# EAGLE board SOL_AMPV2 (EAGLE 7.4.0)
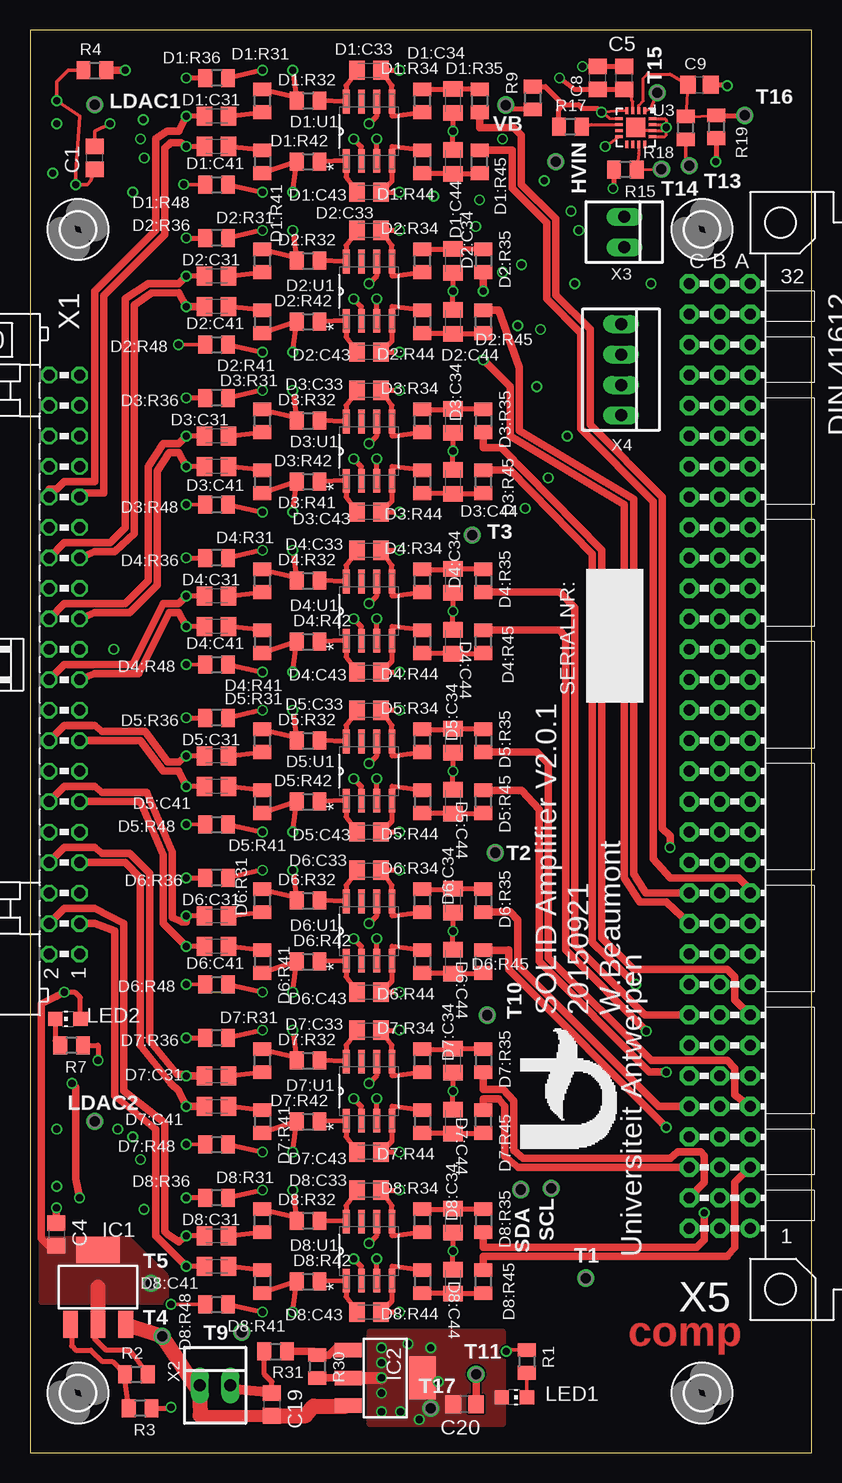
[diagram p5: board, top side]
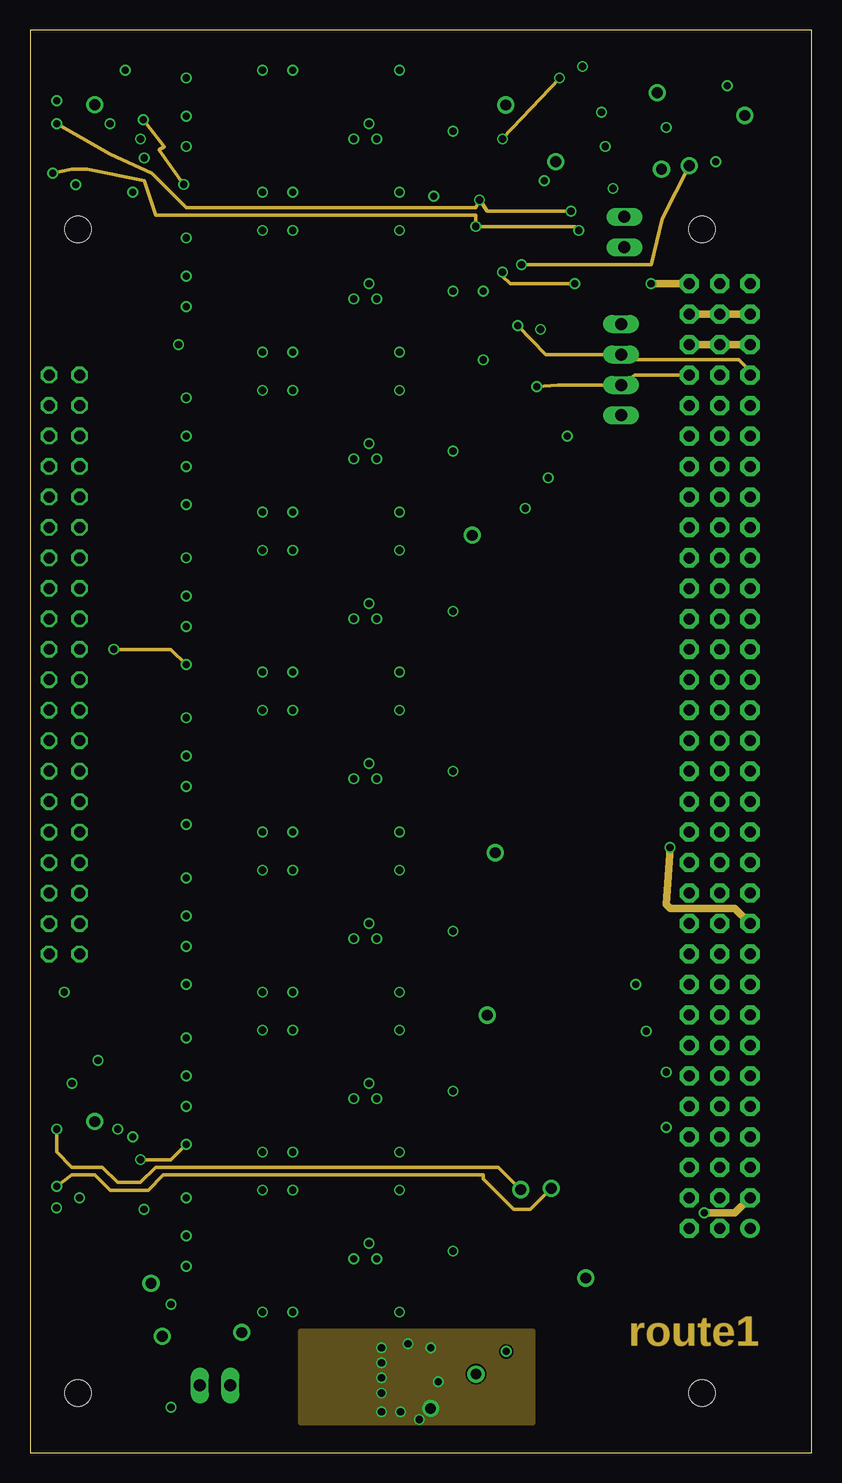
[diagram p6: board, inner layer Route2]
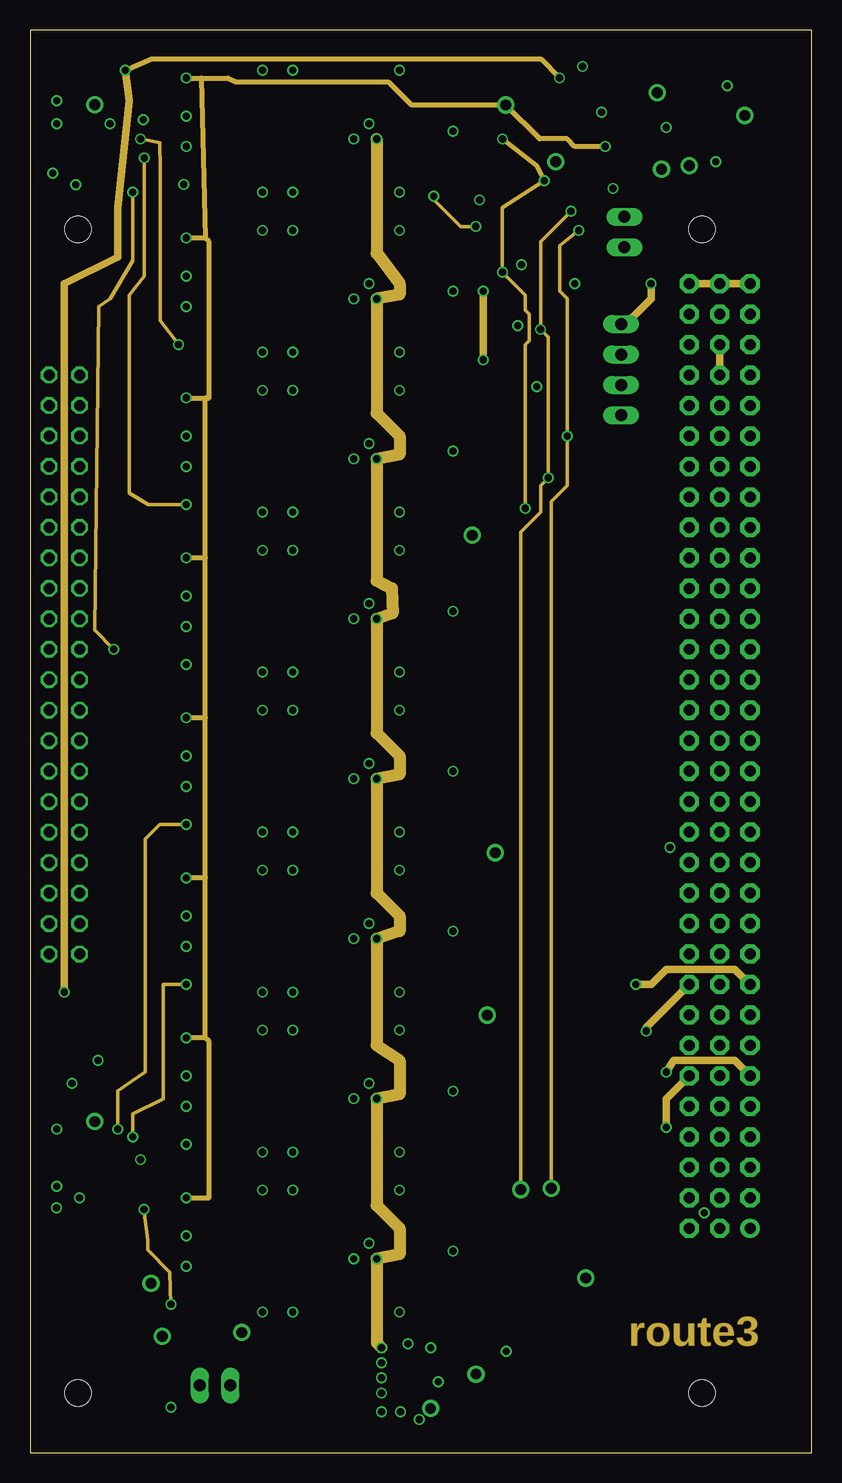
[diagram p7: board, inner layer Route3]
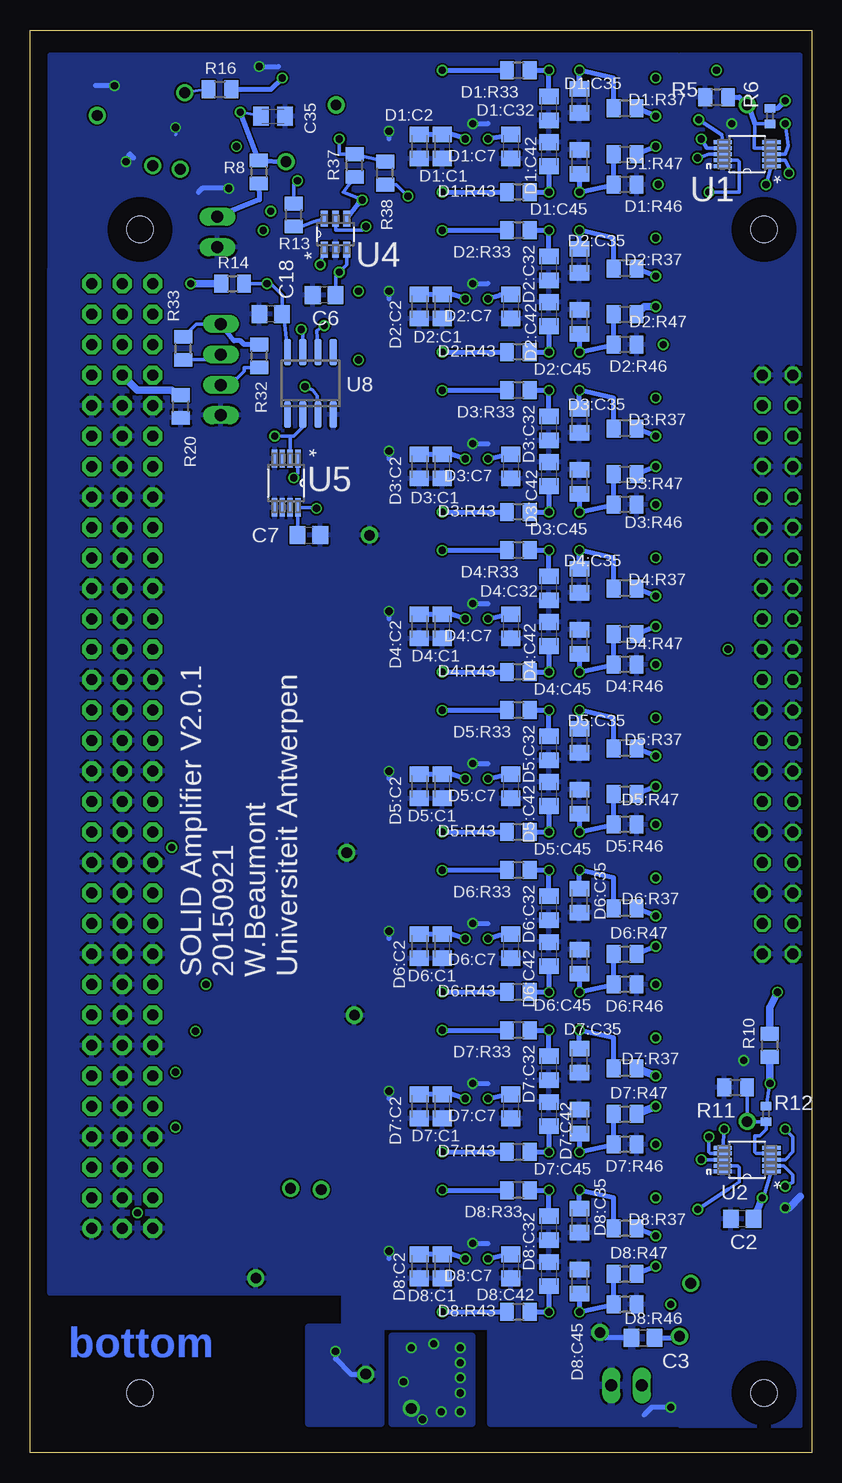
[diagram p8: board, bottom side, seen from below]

Size 65.15 x 118.62 mm. Coordinates in mm from the lower left corner, seen from the top.
Outline: 0,0 65.15,0 65.15,118.62 0,118.62 0,0
Copper layers (1+2*3+16): Top 0.018mm / dielectric 0.36mm / Route2 0.035mm / dielectric 0.71mm / Route3 0.035mm / dielectric 0.36mm / Bottom 0.018mm
Design rules "eC_4Layer_PClass6_BaseCopperO18-I35_eCDefault": minimum track width 0.15mm, minimum drill 0.35mm, track to track 0.15mm, track to pad 0.15mm, pad to pad 0.15mm, via to via 0.15mm, smd to smd 0mil, copper to edge 0.25mm, drill to drill 0.35mm, minimum pad ring 0.175mm, minimum via ring 0.125mm, stop-mask expansion 0mil, vias tented up to drill 0.45mm, thermal gap 0.2mm

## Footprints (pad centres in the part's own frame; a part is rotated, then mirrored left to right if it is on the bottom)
C0805 = smd 1.3 x 1.5: 1 -0.95,0; 2 0.95,0
C0805K = smd 1.3 x 1.6: 1 -1,0; 2 1,0
R0805H = smd 1.143 x 1.5: 1 -0.95,0; 2 0.95,0
SOIC127P600X175-8N = smd 1.981 x 0.559: 1 -2.464,1.905; 2 -2.464,0.635; 3 -2.464,-0.635; 4 -2.464,-1.905; 5 2.464,-1.905; 6 2.464,-0.635; 7 2.464,0.635; 8 2.464,1.905
2,1 = hole 2.2: 0,0
UA_P1-13 = drill 0.9 pad 1.422: TP 0,0
SOT223 = smd 1.219 x 2.235: 1 -2.311,-3.099; 2 0,-3.099; 3 2.311,-3.099 | smd 3.6 x 2.2: 4 0,3.099
CHIP-LED0805 = smd 1.2 x 1.2: A 0,-1.05; C 0,1.05
R0402 = smd 0.7 x 0.9: 1 -0.65,0; 2 0.65,0
SOP50P490X110-10N = smd 1.524 x 0.33: 1 -2.032,0.991; 2 -2.032,0.508; 3 -2.032,0; 4 -2.032,-0.508; 5 -2.032,-0.991; 6 2.032,-0.991; 7 2.032,-0.508; 8 2.032,0; 9 2.032,0.508; 10 2.032,0.991
LFCSP_LQ-16_MANSOL = smd 0.61 x 0.25: 1 -1.405,0.75; 2 -1.405,0.25; 3 -1.405,-0.25; 4 -1.405,-0.75; 9 1.405,-0.75; 10 1.405,-0.25; 11 1.405,0.25; 12 1.405,0.75 | smd 0.25 x 0.61: 5 -0.75,-1.405; 6 -0.25,-1.405; 7 0.25,-1.405; 8 0.75,-1.405; 13 0.75,1.405; 14 0.25,1.405; 15 -0.25,1.405; 16 -0.75,1.405 | smd 1.6 x 1.6: EXP 0,0
SOT95P270X145-6N = smd 1.321 x 0.559: 1 -1.295,0.94; 2 -1.295,0; 3 -1.295,-0.94; 4 1.295,-0.94; 5 1.295,0; 6 1.295,0.94
SOP65P490X110-8N = smd 1.524 x 0.457: 1 -2.032,0.965; 2 -2.032,0.33; 3 -2.032,-0.33; 4 -2.032,-0.965; 5 2.032,-0.965; 6 2.032,-0.33; 7 2.032,0.33; 8 2.032,0.965
SO8 = smd 0.6 x 2.2: 1 -1.905,-2.6; 2 -0.635,-2.6; 3 0.635,-2.6; 4 1.905,-2.6; 5 1.905,2.6; 6 0.635,2.6; 7 -0.635,2.6; 8 -1.905,2.6
ML40L = drill 0.914 octagon: 1 -24.13,-1.27; 2 -24.13,1.27; 3 -21.59,-1.27; 4 -21.59,1.27; 5 -19.05,-1.27; 6 -19.05,1.27; 7 -16.51,-1.27; 8 -16.51,1.27; 9 -13.97,-1.27; 10 -13.97,1.27; 11 -11.43,-1.27; 12 -11.43,1.27; 13 -8.89,-1.27; 14 -8.89,1.27; 15 -6.35,-1.27; 16 -6.35,1.27; 17 -3.81,-1.27; 18 -3.81,1.27; 19 -1.27,-1.27; 20 -1.27,1.27; 21 1.27,-1.27; 22 1.27,1.27; 23 3.81,-1.27; 24 3.81,1.27; 25 6.35,-1.27; 26 6.35,1.27; 27 8.89,-1.27; 28 8.89,1.27; 29 11.43,-1.27; 30 11.43,1.27; 31 13.97,-1.27; 32 13.97,1.27; 33 16.51,-1.27; 34 16.51,1.27; 35 19.05,-1.27; 36 19.05,1.27; 37 21.59,-1.27; 38 21.59,1.27; 39 24.13,-1.27; 40 24.13,1.27
22-23-2021 = drill 1 long: 1 -1.27,0; 2 1.27,0
22-23-2041 = drill 1 long: 1 -3.81,0; 2 -1.27,0; 3 1.27,0; 4 3.81,0
DIN41612_96RC = drill 0.914 pad 1.6: A1 2.54,-39.37 | drill 0.914 pad 1.6 octagon: A2 2.54,-36.83; A3 2.54,-34.29; A4 2.54,-31.75; A5 2.54,-29.21; A6 2.54,-26.67; A7 2.54,-24.13; A8 2.54,-21.59; A9 2.54,-19.05; A10 2.54,-16.51; A11 2.54,-13.97; A12 2.54,-11.43; A13 2.54,-8.89; A14 2.54,-6.35; A15 2.54,-3.81; A16 2.54,-1.27; A17 2.54,1.27; A18 2.54,3.81; A19 2.54,6.35; A20 2.54,8.89; A21 2.54,11.43; A22 2.54,13.97; A23 2.54,16.51; A24 2.54,19.05; A25 2.54,21.59; A26 2.54,24.13; A27 2.54,26.67; A28 2.54,29.21; A29 2.54,31.75; A30 2.54,34.29; A31 2.54,36.83; A32 2.54,39.37; B1 0,-39.37; B2 0,-36.83; B3 0,-34.29; B4 0,-31.75; B5 0,-29.21; B6 0,-26.67; B7 0,-24.13; B8 0,-21.59; B9 0,-19.05; B10 0,-16.51; B11 0,-13.97; B12 0,-11.43; B13 0,-8.89; B14 0,-6.35; B15 0,-3.81; B16 0,-1.27; B17 0,1.27; B18 0,3.81; B19 0,6.35; B20 0,8.89; B21 0,11.43; B22 0,13.97; B23 0,16.51; B24 0,19.05; B25 0,21.59; B26 0,24.13; B27 0,26.67; B28 0,29.21; B29 0,31.75; B30 0,34.29; B31 0,36.83; B32 0,39.37; C1 -2.54,-39.37; C2 -2.54,-36.83; C3 -2.54,-34.29; C4 -2.54,-31.75; C5 -2.54,-29.21; C6 -2.54,-26.67; C7 -2.54,-24.13; C8 -2.54,-21.59; C9 -2.54,-19.05; C10 -2.54,-16.51; C11 -2.54,-13.97; C12 -2.54,-11.43; C13 -2.54,-8.89; C14 -2.54,-6.35; C15 -2.54,-3.81; C16 -2.54,-1.27; C17 -2.54,1.27; C18 -2.54,3.81; C19 -2.54,6.35; C20 -2.54,8.89; C21 -2.54,11.43; C22 -2.54,13.97; C23 -2.54,16.51; C24 -2.54,19.05; C25 -2.54,21.59; C26 -2.54,24.13; C27 -2.54,26.67; C28 -2.54,29.21; C29 -2.54,31.75; C30 -2.54,34.29; C31 -2.54,36.83; C32 -2.54,39.37

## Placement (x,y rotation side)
C1  10u  [C0805]  5.4,107.95 90 top
C2  10u  [C0805]  5.79,19.51 180 bottom
C3  10uF  [C0805]  14.06,9.59 0 bottom
C4  10uF  [C0805]  2.21,18.22 270 top
C5  10n  [C0805]  49.53,114.62 90 top
C6  10n  [C0805]  40.64,96.52 180 bottom
C7  10n  [C0805]  41.91,76.52 0 bottom
C8  100n  [C0805]  47.31,114.62 90 top
C9  10n  [C0805]  55.78,114.05 0 top
C18  10n  [C0805]  45.09,94.93 180 bottom
C19  10uF  [C0805]  20.16,4.05 270 top
C20  10uF  [C0805]  36.22,4.05 180 top
C35  100nF /100V  [C0805K]  44.9,111.42 0 bottom
D1:C1  100n  [C0805K]  30.8,108.9 90 bottom
D1:C2  10n  [C0805K]  32.7,108.9 90 bottom
D1:C7  10n  [C0805K]  25.08,108.9 270 bottom
D1:C31  4.4n/100V  [C0805K]  15.56,111.44 180 top
D1:C32  152p  [C0805K]  21.91,112.08 90 bottom
D1:C33  21p  [C0805K]  28.26,115.25 0 top
D1:C34  x  [C0805K]  35.24,112.71 90 top
D1:C35  100nF /100V  [C0805K]  19.37,112.71 270 bottom
D1:C41  4.4n  [C0805K]  15.56,108.9 180 top
D1:C42  152p  [C0805K]  21.91,108.27 270 bottom
D1:C43  21p  [C0805K]  28.26,105.09 0 top
D1:C44  x  [C0805K]  35.24,107.63 270 top
D1:C45  100nF /100V  [C0805K]  19.37,107.63 90 bottom
D1:R31  27  [R0805H]  19.37,112.71 90 top
D1:R32  24  [R0805H]  23.18,112.71 0 top
D1:R33  3K  [R0805H]  24.45,115.25 180 bottom
D1:R34  1  [R0805H]  32.7,112.71 90 top
D1:R35  1  [R0805H]  37.47,112.71 270 top
D1:R36  10K  [R0805H]  15.56,114.62 180 top
D1:R37  100K  [R0805H]  15.56,112.08 180 bottom
D1:R41  27  [R0805H]  19.37,107.63 270 top
D1:R42  24  [R0805H]  23.18,107.63 0 top
D1:R43  3K  [R0805H]  24.45,105.09 180 bottom
D1:R44  1  [R0805H]  32.7,107.63 270 top
D1:R45  1  [R0805H]  37.47,107.63 90 top
D1:R46  10K  [R0805H]  15.56,105.73 180 bottom
D1:R47  100K  [R0805H]  15.56,108.27 0 bottom
D1:R48  470  [R0805H]  15.56,105.73 0 top
D1:U1  AD8132ARZ  [SOIC127P600X175-8N]  28.26,110.17 90 top
D2:C1  100n  [C0805K]  30.8,95.57 90 bottom
D2:C2  10n  [C0805K]  32.7,95.57 90 bottom
D2:C7  10n  [C0805K]  25.08,95.57 270 bottom
D2:C31  4.4n/100V  [C0805K]  15.56,98.11 180 top
D2:C32  152p  [C0805K]  21.91,98.74 90 bottom
D2:C33  21p  [C0805K]  28.26,101.92 0 top
D2:C34  x  [C0805K]  35.24,99.38 90 top
D2:C35  100nF /100V  [C0805K]  19.37,99.38 270 bottom
D2:C41  4.4n  [C0805K]  15.56,95.57 180 top
D2:C42  152p  [C0805K]  21.91,94.93 270 bottom
D2:C43  21p  [C0805K]  28.26,91.76 0 top
D2:C44  x  [C0805K]  35.24,94.3 270 top
D2:C45  100nF /100V  [C0805K]  19.37,94.3 90 bottom
D2:R31  27  [R0805H]  19.37,99.38 90 top
D2:R32  24  [R0805H]  23.18,99.38 0 top
D2:R33  3K  [R0805H]  24.45,101.92 180 bottom
D2:R34  1  [R0805H]  32.7,99.38 90 top
D2:R35  1  [R0805H]  37.78,99.38 270 top
D2:R36  10K  [R0805H]  15.56,101.28 180 top
D2:R37  100K  [R0805H]  15.56,98.74 180 bottom
D2:R41  27  [R0805H]  19.37,94.3 270 top
D2:R42  24  [R0805H]  23.18,94.3 0 top
D2:R43  3K  [R0805H]  24.45,91.76 180 bottom
D2:R44  1  [R0805H]  32.7,94.3 270 top
D2:R45  1  [R0805H]  37.78,94.3 90 top
D2:R46  10K  [R0805H]  15.56,92.39 180 bottom
D2:R47  100K  [R0805H]  15.56,94.93 0 bottom
D2:R48  470  [R0805H]  15.56,92.39 0 top
D2:U1  AD8132ARZ  [SOIC127P600X175-8N]  28.26,96.84 90 top
D3:C1  100n  [C0805K]  30.8,82.23 90 bottom
D3:C2  10n  [C0805K]  32.7,82.23 90 bottom
D3:C7  10n  [C0805K]  25.08,82.23 270 bottom
D3:C31  4.4n/100V  [C0805K]  15.56,84.77 180 top
D3:C32  152p  [C0805K]  21.91,85.41 90 bottom
D3:C33  21p  [C0805K]  28.26,88.58 0 top
D3:C34  x  [C0805K]  35.24,86.04 90 top
D3:C35  100nF /100V  [C0805K]  19.37,86.04 270 bottom
D3:C41  4.4n  [C0805K]  15.56,82.23 180 top
D3:C42  152p  [C0805K]  21.91,81.6 270 bottom
D3:C43  21p  [C0805K]  28.26,78.42 0 top
D3:C44  x  [C0805K]  35.24,80.96 270 top
D3:C45  100nF /100V  [C0805K]  19.37,80.96 90 bottom
D3:R31  27  [R0805H]  19.37,86.04 90 top
D3:R32  24  [R0805H]  23.18,86.04 0 top
D3:R33  3K  [R0805H]  24.45,88.58 180 bottom
D3:R34  1  [R0805H]  32.7,86.04 90 top
D3:R35  1  [R0805H]  37.78,86.04 270 top
D3:R36  10K  [R0805H]  15.56,87.95 180 top
D3:R37  100K  [R0805H]  15.56,85.41 180 bottom
D3:R41  27  [R0805H]  19.37,80.96 270 top
D3:R42  24  [R0805H]  23.18,80.96 0 top
D3:R43  3K  [R0805H]  24.45,78.42 180 bottom
D3:R44  1  [R0805H]  32.7,80.96 270 top
D3:R45  1  [R0805H]  37.78,80.96 90 top
D3:R46  10K  [R0805H]  15.56,79.06 180 bottom
D3:R47  100K  [R0805H]  15.56,81.6 0 bottom
D3:R48  470  [R0805H]  15.56,79.06 0 top
D3:U1  AD8132ARZ  [SOIC127P600X175-8N]  28.26,83.5 90 top
D4:C1  100n  [C0805K]  30.8,68.9 90 bottom
D4:C2  10n  [C0805K]  32.7,68.9 90 bottom
D4:C7  10n  [C0805K]  25.08,68.9 270 bottom
D4:C31  4.4n/100V  [C0805K]  15.56,71.44 180 top
D4:C32  152p  [C0805K]  21.91,72.07 90 bottom
D4:C33  21p  [C0805K]  28.26,75.25 0 top
D4:C34  x  [C0805K]  35.24,72.71 90 top
D4:C35  100nF /100V  [C0805K]  19.37,72.71 270 bottom
D4:C41  4.4n  [C0805K]  15.56,68.9 180 top
D4:C42  152p  [C0805K]  21.91,68.26 270 bottom
D4:C43  21p  [C0805K]  28.26,65.09 0 top
D4:C44  x  [C0805K]  35.24,67.63 270 top
D4:C45  100nF /100V  [C0805K]  19.37,67.63 90 bottom
D4:R31  27  [R0805H]  19.37,72.71 90 top
D4:R32  24  [R0805H]  23.18,72.71 0 top
D4:R33  3K  [R0805H]  24.45,75.25 180 bottom
D4:R34  1  [R0805H]  32.7,72.71 90 top
D4:R35  1  [R0805H]  37.78,72.71 270 top
D4:R36  10K  [R0805H]  15.56,74.61 180 top
D4:R37  100K  [R0805H]  15.56,72.07 180 bottom
D4:R41  27  [R0805H]  19.37,67.63 270 top
D4:R42  24  [R0805H]  23.18,67.63 0 top
D4:R43  3K  [R0805H]  24.45,65.09 180 bottom
D4:R44  1  [R0805H]  32.7,67.63 270 top
D4:R45  1  [R0805H]  37.78,67.63 90 top
D4:R46  10K  [R0805H]  15.56,65.72 180 bottom
D4:R47  100K  [R0805H]  15.56,68.26 0 bottom
D4:R48  470  [R0805H]  15.56,65.72 0 top
D4:U1  AD8132ARZ  [SOIC127P600X175-8N]  28.26,70.17 90 top
D5:C1  100n  [C0805K]  30.8,55.56 90 bottom
D5:C2  10n  [C0805K]  32.7,55.56 90 bottom
D5:C7  10n  [C0805K]  25.08,55.56 270 bottom
D5:C31  4.4n/100V  [C0805K]  15.56,58.1 180 top
D5:C32  152p  [C0805K]  21.91,58.74 90 bottom
D5:C33  21p  [C0805K]  28.26,61.91 0 top
D5:C34  x  [C0805K]  35.24,59.37 90 top
D5:C35  100nF /100V  [C0805K]  19.37,59.37 270 bottom
D5:C41  4.4n  [C0805K]  15.56,55.56 180 top
D5:C42  152p  [C0805K]  21.91,54.93 270 bottom
D5:C43  21p  [C0805K]  28.26,51.75 0 top
D5:C44  x  [C0805K]  35.24,54.29 270 top
D5:C45  100nF /100V  [C0805K]  19.37,54.29 90 bottom
D5:R31  27  [R0805H]  19.37,59.37 90 top
D5:R32  24  [R0805H]  23.18,59.37 0 top
D5:R33  3K  [R0805H]  24.45,61.91 180 bottom
D5:R34  1  [R0805H]  32.7,59.37 90 top
D5:R35  1  [R0805H]  37.78,59.37 270 top
D5:R36  10K  [R0805H]  15.56,61.28 180 top
D5:R37  100K  [R0805H]  15.56,58.74 180 bottom
D5:R41  27  [R0805H]  19.37,54.29 270 top
D5:R42  24  [R0805H]  23.18,54.29 0 top
D5:R43  3K  [R0805H]  24.45,51.75 180 bottom
D5:R44  1  [R0805H]  32.7,54.29 270 top
D5:R45  1  [R0805H]  37.78,54.29 90 top
D5:R46  10K  [R0805H]  15.56,52.39 180 bottom
D5:R47  100K  [R0805H]  15.56,54.93 0 bottom
D5:R48  470  [R0805H]  15.56,52.39 0 top
D5:U1  AD8132ARZ  [SOIC127P600X175-8N]  28.26,56.83 90 top
D6:C1  100n  [C0805K]  30.8,42.23 90 bottom
D6:C2  10n  [C0805K]  32.7,42.23 90 bottom
D6:C7  10n  [C0805K]  25.08,42.23 270 bottom
D6:C31  4.4n/100V  [C0805K]  15.56,44.77 180 top
D6:C32  152p  [C0805K]  21.91,45.4 90 bottom
D6:C33  21p  [C0805K]  28.26,48.58 0 top
D6:C34  x  [C0805K]  35.24,46.04 90 top
D6:C35  100nF /100V  [C0805K]  19.37,46.04 270 bottom
D6:C41  4.4n  [C0805K]  15.56,42.23 180 top
D6:C42  152p  [C0805K]  21.91,41.59 270 bottom
D6:C43  21p  [C0805K]  28.26,38.42 0 top
D6:C44  x  [C0805K]  35.24,40.96 270 top
D6:C45  100nF /100V  [C0805K]  19.37,40.96 90 bottom
D6:R31  27  [R0805H]  19.37,46.04 90 top
D6:R32  24  [R0805H]  23.18,46.04 0 top
D6:R33  3K  [R0805H]  24.45,48.58 180 bottom
D6:R34  1  [R0805H]  32.7,46.04 90 top
D6:R35  1  [R0805H]  37.78,46.04 270 top
D6:R36  10K  [R0805H]  15.56,47.94 180 top
D6:R37  100K  [R0805H]  15.56,45.4 180 bottom
D6:R41  27  [R0805H]  19.37,40.96 270 top
D6:R42  24  [R0805H]  23.18,40.96 0 top
D6:R43  3K  [R0805H]  24.45,38.42 180 bottom
D6:R44  1  [R0805H]  32.7,40.96 270 top
D6:R45  1  [R0805H]  37.78,40.96 90 top
D6:R46  10K  [R0805H]  15.56,39.05 180 bottom
D6:R47  100K  [R0805H]  15.56,41.59 0 bottom
D6:R48  470  [R0805H]  15.56,39.05 0 top
D6:U1  AD8132ARZ  [SOIC127P600X175-8N]  28.26,43.5 90 top
D7:C1  100n  [C0805K]  30.8,28.89 90 bottom
D7:C2  10n  [C0805K]  32.7,28.89 90 bottom
D7:C7  10n  [C0805K]  25.08,28.89 270 bottom
D7:C31  4.4n/100V  [C0805K]  15.56,31.43 180 top
D7:C32  152p  [C0805K]  21.91,32.07 90 bottom
D7:C33  21p  [C0805K]  28.26,35.24 0 top
D7:C34  x  [C0805K]  35.24,32.7 90 top
D7:C35  100nF /100V  [C0805K]  19.37,32.7 270 bottom
D7:C41  4.4n  [C0805K]  15.56,28.89 180 top
D7:C42  152p  [C0805K]  21.91,28.26 270 bottom
D7:C43  21p  [C0805K]  28.26,25.08 0 top
D7:C44  x  [C0805K]  35.24,27.62 270 top
D7:C45  100nF /100V  [C0805K]  19.37,27.62 90 bottom
D7:R31  27  [R0805H]  19.37,32.7 90 top
D7:R32  24  [R0805H]  23.18,32.7 0 top
D7:R33  3K  [R0805H]  24.45,35.24 180 bottom
D7:R34  1  [R0805H]  32.7,32.7 90 top
D7:R35  1  [R0805H]  37.78,32.7 270 top
D7:R36  10K  [R0805H]  15.56,34.61 180 top
D7:R37  100K  [R0805H]  15.56,32.07 180 bottom
D7:R41  27  [R0805H]  19.37,27.62 270 top
D7:R42  24  [R0805H]  23.18,27.62 0 top
D7:R43  3K  [R0805H]  24.45,25.08 180 bottom
D7:R44  1  [R0805H]  32.7,27.62 270 top
D7:R45  1  [R0805H]  37.78,27.62 90 top
D7:R46  10K  [R0805H]  15.56,25.72 180 bottom
D7:R47  100K  [R0805H]  15.56,28.26 0 bottom
D7:R48  470  [R0805H]  15.56,25.72 0 top
D7:U1  AD8132ARZ  [SOIC127P600X175-8N]  28.26,30.16 90 top
D8:C1  100n  [C0805K]  30.8,15.56 90 bottom
D8:C2  10n  [C0805K]  32.7,15.56 90 bottom
D8:C7  10n  [C0805K]  25.08,15.56 270 bottom
D8:C31  4.4n/100V  [C0805K]  15.56,18.1 180 top
D8:C32  152p  [C0805K]  21.91,18.73 90 bottom
D8:C33  21p  [C0805K]  28.26,21.91 0 top
D8:C34  x  [C0805K]  35.24,19.37 90 top
D8:C35  100nF /100V  [C0805K]  19.37,19.37 270 bottom
D8:C41  4.4n  [C0805K]  15.56,15.56 180 top
D8:C42  152p  [C0805K]  21.91,14.92 270 bottom
D8:C43  21p  [C0805K]  28.26,11.75 0 top
D8:C44  x  [C0805K]  35.24,14.29 270 top
D8:C45  100nF /100V  [C0805K]  19.37,14.29 90 bottom
D8:R31  27  [R0805H]  19.37,19.37 90 top
D8:R32  24  [R0805H]  23.18,19.37 0 top
D8:R33  3K  [R0805H]  24.45,21.91 180 bottom
D8:R34  1  [R0805H]  32.7,19.37 90 top
D8:R35  1  [R0805H]  37.78,19.37 270 top
D8:R36  10K  [R0805H]  15.56,21.27 180 top
D8:R37  100K  [R0805H]  15.56,18.73 180 bottom
D8:R41  27  [R0805H]  19.37,14.29 270 top
D8:R42  24  [R0805H]  23.18,14.29 0 top
D8:R43  3K  [R0805H]  24.45,11.75 180 bottom
D8:R44  1  [R0805H]  32.7,14.29 270 top
D8:R45  1  [R0805H]  37.78,14.29 90 top
D8:R46  10K  [R0805H]  15.56,12.38 180 bottom
D8:R47  100K  [R0805H]  15.56,14.92 0 bottom
D8:R48  470  [R0805H]  15.56,12.38 0 top
D8:U1  AD8132ARZ  [SOIC127P600X175-8N]  28.26,16.83 90 top
H1  [2,1]  4,5 0 top
H2  [2,1]  56,5 0 top
H3  [2,1]  4,102 0 top
H4  [2,1]  56,102 0 top
HVIN  UA_TPPAD1-13  [UA_P1-13]  43.81,107.63 0 top
IC1  LM1117  [SOT223]  5.67,13.82 0 top
IC2  LM1117  [SOT223]  29.61,6.26 270 top
LDAC1  UA_TPPAD1-13  [UA_P1-13]  5.4,112.39 0 top
LDAC2  UA_TPPAD1-13  [UA_P1-13]  5.4,27.62 0 top
LED1  HSMY-C170  [CHIP-LED0805]  40.36,4.64 270 top
LED2  HSMY-C170  [CHIP-LED0805]  3.15,36.18 90 top
M1  [UA]  45.09,29.21 90 top
R1  1K  [R0805H]  41.4,7.63 270 top
R2  330E  [R0805H]  8.86,6.57 0 top
R3  1K  [R0805H]  9.17,3.73 180 top
R4  10E  [R0805H]  5.4,115.25 0 top
R5  4.7K  [R0805H]  7.94,113.03 0 bottom
R6  NC  [R0402]  3.49,111.44 90 bottom
R7  1K  [R0805H]  3.47,33.97 180 top
R8  1K  [R0805H]  46.09,106.79 270 bottom
R9  NC  [R0805H]  41.91,112.95 90 top
R10  10  [R0805H]  3.49,33.97 90 bottom
R11  4.7K  [R0805H]  6.35,30.48 0 bottom
R12  NC  [R0402]  3.81,28.26 90 bottom
R13  4K7  [R0805H]  43.18,103.19 90 bottom
R14  NC  [R0805H]  48.26,97.47 0 bottom
R15  27K  [R0805H]  49.62,106.96 180 top
R16  1K  [R0805H]  49.32,113.67 0 bottom
R17  NC  [R0805H]  45.03,110.57 0 top
R18  1K  [R0805H]  54.65,110.45 90 top
R19  2.4K  [R0805H]  57.19,110.54 270 top
R20  0  [R0805H]  52.58,87.24 90 bottom
R30  330E  [R0805H]  23.94,7.2 270 top
R31  1K  [R0805H]  20.47,8.46 0 top
R32  4K7  [R0805H]  46.04,91.44 90 bottom
R33  4K7  [R0805H]  52.39,92.08 90 bottom
R37  4K7  [R0805H]  38.1,107.31 90 bottom
R38  4K7  [R0805H]  35.56,106.68 90 bottom
SCL  UA_TPPAD1-13  [UA_P1-13]  43.44,22.06 0 top
SDA  UA_TPPAD1-13  [UA_P1-13]  40.89,21.95 0 top
T1  UA_TPPAD1-13  [UA_P1-13]  46.32,14.57 0 top
T2  UA_TPPAD1-13  [UA_P1-13]  38.76,50.04 0 top
T3  UA_TPPAD1-13  [UA_P1-13]  36.86,76.5 0 top
T4  UA_TPPAD1-13  [UA_P1-13]  11.03,9.73 0 top
T5  UA_TPPAD1-13  [UA_P1-13]  10.08,14.13 0 top
T9  UA_TPPAD1-13  [UA_P1-13]  17.65,10.04 0 top
T10  UA_TPPAD1-13  [UA_P1-13]  38.11,36.49 0 top
T11  UA_TPPAD1-13  [UA_P1-13]  37.17,6.57 0 top
T13  UA_TPPAD1-13  [UA_P1-13]  54.93,107.31 0 top
T14  UA_TPPAD1-13  [UA_P1-13]  52.62,107.01 0 top
T15  UA_TPPAD1-13  [UA_P1-13]  52.26,113.39 0 top
T16  UA_TPPAD1-13  [UA_P1-13]  59.56,111.5 0 top
T17  UA_TPPAD1-13  [UA_P1-13]  33.38,3.71 0 top
U1  MCP4728-E/UN  [SOP50P490X110-10N]  5.4,108.27 180 bottom
U2  MCP4728-E/UN  [SOP50P490X110-10N]  5.4,24.45 180 bottom
U3  ADL5317  [LFCSP_LQ-16_MANSOL]  50.48,110.49 270 top
U4  MCP4725A0T-E/CH  [SOT95P270X145-6N]  39.69,101.6 90 bottom
U5  MCP9808-E/MS  [SOP65P490X110-8N]  43.8,80.85 270 bottom
U8  P82B715TD  [SO8]  41.79,89.16 0 bottom
VB  UA_TPPAD1-13  [UA_P1-13]  39.64,112.37 0 top
X1  40pin  [ML40L]  2.86,65.72 90 top
X2  22-23-2021  [22-23-2021]  15.44,5.63 0 top
X3  22-23-2021  [22-23-2021]  49.53,101.78 270 top
X4  22-23-2041  [22-23-2041]  49.25,90.3 270 top
X5  DIN41612_ABC_96_R  [DIN41612_96RC]  57.47,58.1 0 top

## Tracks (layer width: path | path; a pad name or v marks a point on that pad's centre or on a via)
BIASSET
  Top 0.254: U3.2 50.72,112.32 51.12,112.71 51.12,114.62 51.44,114.94 53.34,114.94 C9.1 R18.2 R19.1
  Top 0.406: R19.1 T16.TP
BIASTRSET  (via drill 0.6)
  Top 0.305: R18.1 54.65,107.6 T13.TP
  Route2 0.305: v40.96,99.06 51.75,99.06 52.7,102.87 T13.TP
  Bottom 0.305: U4.1 40.63,100.32 40.64,100.33 v40.96,99.06
D1:AOUT+  (via drill 0.6)
  Top 0.406: v30.8,105.09 D1:C43.2 30.16,106 D1:U1.4 30.16,108.9 D1:R44.1
  Bottom 0.406: v30.8,105.09 D1:R43.2
D1:AOUT-  (via drill 0.6)
  Top 0.406: D1:R34.1 30.16,111.44 D1:U1.5 30.16,113.98 D1:C33.2 v30.8,115.25
  Bottom 0.406: v30.8,115.25 D1:R33.2
D1:FB+  (via drill 0.6)
  Top 0.406: v21.91,115.25 D1:R32.1 D1:C32.2 D1:R31.2
  Bottom 0.406: D1:R33.1 v21.91,115.25 D1:C32.2
D1:FB-  (via drill 0.6)
  Top 0.406: v21.91,105.09 D1:R42.1 D1:R41.2
  Bottom 0.406: D1:R43.1 v21.91,105.09 D1:C42.2
D1:N$1
  Top 0.406: D1:R34.2 35.24,113.66 D1:C34.2 37.78,113.71 D1:R35.1
D1:N$2  (via drill 0.6)
  Top 0.406: D1:U1.2 27.62,108.9 v26.99,109.54
  Bottom 0.406: v26.99,109.54 25.35,109.86 D1:C7.1
D1:N$3
  Top 0.406: D1:R44.2 35.24,106.68 D1:C44.2 37.78,106.63 D1:R45.1
D1:N$4
  Top 0.406: D1:R42.2 D1:U1.1 26.35,106.36 D1:C43.1
D1:N$5
  Top 0.406: D1:C33.1 26.35,113.98 D1:U1.8 D1:R32.2
D1:N$10
  Top 0.406: D1:R41.1 D1:C41.1
D1:R31
  Top 0.406: D1:C31.1 D1:R31.1
D1:VB+  (via drill 0.6)
  Top 0.406: v19.37,115.25 D1:R36.1
  Bottom 0.406: D1:C35.1 v19.37,115.25 D1:R36.1 D1:R37.2
D1:VB-  (via drill 0.6)
  Top 0.406: D1:R46.2 v19.37,105.09
  Bottom 0.406: D1:R47.1 D1:R46.2 v19.37,105.09 D1:C45.1
D2:AOUT+  (via drill 0.6)
  Top 0.406: v30.8,91.76 D2:C43.2 30.16,92.66 D2:U1.4 30.16,95.57 D2:R44.1
  Bottom 0.406: v30.8,91.76 D2:R43.2
D2:AOUT-  (via drill 0.6)
  Top 0.406: D2:R34.1 30.16,98.11 D2:U1.5 30.16,100.65 D2:C33.2 v30.8,101.92
  Bottom 0.406: v30.8,101.92 D2:R33.2
D2:FB+  (via drill 0.6)
  Top 0.406: v21.91,101.92 D2:R32.1 D2:C32.2 D2:R31.2
  Bottom 0.406: D2:R33.1 v21.91,101.92 D2:C32.2
D2:FB-  (via drill 0.6)
  Top 0.406: v21.91,91.76 D2:R42.1 D2:R41.2
  Bottom 0.406: D2:R43.1 v21.91,91.76 D2:C42.2
D2:N$1
  Top 0.406: D2:R34.2 35.24,100.33 D2:C34.2 37.78,100.38 D2:R35.1
D2:N$2  (via drill 0.6)
  Top 0.406: D2:U1.2 27.62,95.57 v26.99,96.2
  Bottom 0.406: v26.99,96.2 25.99,96.52 D2:C7.1
D2:N$3
  Top 0.406: D2:R44.2 35.24,93.35 D2:C44.2 37.78,93.3 D2:R45.1
D2:N$4
  Top 0.406: D2:R42.2 D2:U1.1 26.35,93.03 D2:C43.1
D2:N$5
  Top 0.406: D2:C33.1 26.35,100.65 D2:U1.8 D2:R32.2
D2:N$10
  Top 0.406: D2:R41.1 D2:C41.1
D2:R31
  Top 0.406: D2:C31.1 D2:R31.1
D2:VB+  (via drill 0.6)
  Top 0.406: v19.37,101.92 D2:R36.1
  Bottom 0.406: D2:C35.1 v19.37,101.92 D2:R36.1 D2:R37.2
D2:VB-  (via drill 0.6)
  Top 0.406: D2:R46.2 v19.37,91.76
  Bottom 0.406: D2:R47.1 D2:R46.2 v19.37,91.76 D2:C45.1
D3:AOUT+  (via drill 0.6)
  Top 0.406: v30.8,78.42 D3:C43.2 30.16,79.33 D3:U1.4 30.16,82.23 D3:R44.1
  Bottom 0.406: v30.8,78.42 D3:R43.2
D3:AOUT-  (via drill 0.6)
  Top 0.406: D3:R34.1 30.16,84.77 D3:U1.5 30.16,87.31 D3:C33.2 v30.8,88.58
  Bottom 0.406: v30.8,88.58 D3:R33.2
D3:FB+  (via drill 0.6)
  Top 0.406: v21.91,88.58 D3:R32.1 D3:C32.2 D3:R31.2
  Bottom 0.406: D3:R33.1 v21.91,88.58 D3:C32.2
D3:FB-  (via drill 0.6)
  Top 0.406: v21.91,78.42 D3:R42.1 D3:R41.2
  Bottom 0.406: D3:R43.1 v21.91,78.42 D3:C42.2
D3:N$1
  Top 0.406: D3:R34.2 35.24,86.99 D3:C34.2 37.78,87.04 D3:R35.1
D3:N$2  (via drill 0.6)
  Top 0.406: D3:U1.2 27.62,82.23 v26.99,82.87
  Bottom 0.406: v26.99,82.87 25.67,83.19 D3:C7.1
D3:N$3
  Top 0.406: D3:R44.2 35.24,80.01 D3:C44.2 37.78,79.96 D3:R45.1
D3:N$4
  Top 0.406: D3:R42.2 D3:U1.1 26.35,79.69 D3:C43.1
D3:N$5
  Top 0.406: D3:C33.1 26.35,87.31 D3:U1.8 D3:R32.2
D3:N$10
  Top 0.406: D3:R41.1 D3:C41.1
D3:R31
  Top 0.406: D3:C31.1 D3:R31.1
D3:VB+  (via drill 0.6)
  Top 0.406: v19.37,88.58 D3:R36.1
  Bottom 0.406: D3:C35.1 v19.37,88.58 D3:R36.1 D3:R37.2
D3:VB-  (via drill 0.6)
  Top 0.406: D3:R46.2 v19.37,78.42
  Bottom 0.406: D3:R47.1 D3:R46.2 v19.37,78.42 D3:C45.1
D4:AOUT+  (via drill 0.6)
  Top 0.406: v30.8,65.09 D4:C43.2 30.16,65.99 D4:U1.4 30.16,68.9 D4:R44.1
  Bottom 0.406: v30.8,65.09 D4:R43.2
D4:AOUT-  (via drill 0.6)
  Top 0.406: D4:R34.1 30.16,71.44 D4:U1.5 30.16,73.98 D4:C33.2 v30.8,75.25
  Bottom 0.406: v30.8,75.25 D4:R33.2
D4:FB+  (via drill 0.6)
  Top 0.406: v21.91,75.25 D4:R32.1 D4:C32.2 D4:R31.2
  Bottom 0.406: D4:R33.1 v21.91,75.25 D4:C32.2
D4:FB-  (via drill 0.6)
  Top 0.406: v21.91,65.09 D4:R42.1 D4:R41.2
  Bottom 0.406: D4:R43.1 v21.91,65.09 D4:C42.2
D4:N$1
  Top 0.406: D4:R34.2 35.24,73.66 D4:C34.2 37.78,73.71 D4:R35.1
D4:N$2  (via drill 0.6)
  Top 0.406: D4:U1.2 27.62,68.9 v26.99,69.53
  Bottom 0.406: v26.99,69.53 25.67,69.85 D4:C7.1
D4:N$3
  Top 0.406: D4:R44.2 35.24,66.68 D4:C44.2 37.78,66.63 D4:R45.1
D4:N$4
  Top 0.406: D4:R42.2 D4:U1.1 26.35,66.36 D4:C43.1
D4:N$5
  Top 0.406: D4:C33.1 26.35,73.98 D4:U1.8 D4:R32.2
D4:N$10
  Top 0.406: D4:R41.1 D4:C41.1
D4:R31
  Top 0.406: D4:C31.1 D4:R31.1
D4:VB+  (via drill 0.6)
  Top 0.406: v19.37,75.25 D4:R36.1
  Bottom 0.406: D4:C35.1 v19.37,75.25 D4:R36.1 D4:R37.2
D4:VB-  (via drill 0.6)
  Top 0.406: D4:R46.2 v19.37,65.09
  Bottom 0.406: D4:R47.1 D4:R46.2 v19.37,65.09 D4:C45.1
D5:AOUT+  (via drill 0.6)
  Top 0.406: v30.8,51.75 D5:C43.2 30.16,52.66 D5:U1.4 30.16,55.56 D5:R44.1
  Bottom 0.406: v30.8,51.75 D5:R43.2
D5:AOUT-  (via drill 0.6)
  Top 0.406: D5:R34.1 30.16,58.1 D5:U1.5 30.16,60.64 D5:C33.2 v30.8,61.91
  Bottom 0.406: v30.8,61.91 D5:R33.2
D5:FB+  (via drill 0.6)
  Top 0.406: v21.91,61.91 D5:R32.1 D5:C32.2 D5:R31.2
  Bottom 0.406: D5:R33.1 v21.91,61.91 D5:C32.2
D5:FB-  (via drill 0.6)
  Top 0.406: v21.91,51.75 D5:R42.1 D5:R41.2
  Bottom 0.406: D5:R43.1 v21.91,51.75 D5:C42.2
D5:N$1
  Top 0.406: D5:R34.2 35.24,60.32 D5:C34.2 37.78,60.37 D5:R35.1
D5:N$2  (via drill 0.6)
  Top 0.406: D5:U1.2 27.62,55.56 v26.99,56.2
  Bottom 0.406: v26.99,56.2 25.67,56.52 D5:C7.1
D5:N$3
  Top 0.406: D5:R44.2 35.24,53.34 D5:C44.2 37.78,53.29 D5:R45.1
D5:N$4
  Top 0.406: D5:R42.2 D5:U1.1 26.35,53.02 D5:C43.1
D5:N$5
  Top 0.406: D5:C33.1 26.35,60.64 D5:U1.8 D5:R32.2
D5:N$10
  Top 0.406: D5:R41.1 D5:C41.1
D5:R31
  Top 0.406: D5:C31.1 D5:R31.1
D5:VB+  (via drill 0.6)
  Top 0.406: v19.37,61.91 D5:R36.1
  Bottom 0.406: D5:C35.1 v19.37,61.91 D5:R36.1 D5:R37.2
D5:VB-  (via drill 0.6)
  Top 0.406: D5:R46.2 v19.37,51.75
  Bottom 0.406: D5:R47.1 D5:R46.2 v19.37,51.75 D5:C45.1
D6:AOUT+  (via drill 0.6)
  Top 0.406: v30.8,38.42 D6:C43.2 30.16,39.32 D6:U1.4 30.16,42.23 D6:R44.1
  Bottom 0.406: v30.8,38.42 D6:R43.2
D6:AOUT-  (via drill 0.6)
  Top 0.406: D6:R34.1 30.16,44.77 D6:U1.5 30.16,47.31 D6:C33.2 v30.8,48.58
  Bottom 0.406: v30.8,48.58 D6:R33.2
D6:FB+  (via drill 0.6)
  Top 0.406: v21.91,48.58 D6:R32.1 D6:C32.2 D6:R31.2
  Bottom 0.406: D6:R33.1 v21.91,48.58 D6:C32.2
D6:FB-  (via drill 0.6)
  Top 0.406: v21.91,38.42 D6:R42.1 D6:R41.2
  Bottom 0.406: D6:R43.1 v21.91,38.42 D6:C42.2
D6:N$1
  Top 0.406: D6:R34.2 35.24,46.99 D6:C34.2 37.78,47.04 D6:R35.1
D6:N$2  (via drill 0.6)
  Top 0.406: D6:U1.2 27.62,42.23 v26.99,42.86
  Bottom 0.406: v26.99,42.86 25.99,43.18 D6:C7.1
D6:N$3
  Top 0.406: D6:R44.2 35.24,40.01 D6:C44.2 37.78,39.96 D6:R45.1
D6:N$4
  Top 0.406: D6:R42.2 D6:U1.1 26.35,39.69 D6:C43.1
D6:N$5
  Top 0.406: D6:C33.1 26.35,47.31 D6:U1.8 D6:R32.2
D6:N$10
  Top 0.406: D6:R41.1 D6:C41.1
D6:R31
  Top 0.406: D6:C31.1 D6:R31.1
D6:VB+  (via drill 0.6)
  Top 0.406: v19.37,48.58 D6:R36.1
  Bottom 0.406: D6:C35.1 v19.37,48.58 D6:R36.1 D6:R37.2
D6:VB-  (via drill 0.6)
  Top 0.406: D6:R46.2 v19.37,38.42
  Bottom 0.406: D6:R47.1 D6:R46.2 v19.37,38.42 D6:C45.1
D7:AOUT+  (via drill 0.6)
  Top 0.406: v30.8,25.08 D7:C43.2 30.16,25.99 D7:U1.4 30.16,28.89 D7:R44.1
  Bottom 0.406: v30.8,25.08 D7:R43.2
D7:AOUT-  (via drill 0.6)
  Top 0.406: D7:R34.1 30.16,31.43 D7:U1.5 30.16,33.97 D7:C33.2 v30.8,35.24
  Bottom 0.406: v30.8,35.24 D7:R33.2
D7:FB+  (via drill 0.6)
  Top 0.406: v21.91,35.24 D7:R32.1 D7:C32.2 D7:R31.2
  Bottom 0.406: D7:R33.1 v21.91,35.24 D7:C32.2
D7:FB-  (via drill 0.6)
  Top 0.406: v21.91,25.08 D7:R42.1 D7:R41.2
  Bottom 0.406: D7:R43.1 v21.91,25.08 D7:C42.2
D7:N$1
  Top 0.406: D7:R34.2 35.24,33.65 D7:C34.2 37.78,33.7 D7:R35.1
D7:N$2  (via drill 0.6)
  Top 0.406: D7:U1.2 27.62,28.89 v26.99,29.53
  Bottom 0.406: v26.99,29.53 25.67,29.84 D7:C7.1
D7:N$3
  Top 0.406: D7:R44.2 35.24,26.67 D7:C44.2 37.78,26.62 D7:R45.1
D7:N$4
  Top 0.406: D7:R42.2 D7:U1.1 26.35,26.35 D7:C43.1
D7:N$5
  Top 0.406: D7:C33.1 26.35,33.97 D7:U1.8 D7:R32.2
D7:N$10
  Top 0.406: D7:R41.1 D7:C41.1
D7:R31
  Top 0.406: D7:C31.1 D7:R31.1
D7:VB+  (via drill 0.6)
  Top 0.406: v19.37,35.24 D7:R36.1
  Bottom 0.406: D7:C35.1 v19.37,35.24 D7:R36.1 D7:R37.2
D7:VB-  (via drill 0.6)
  Top 0.406: D7:R46.2 v19.37,25.08
  Bottom 0.406: D7:R47.1 D7:R46.2 v19.37,25.08 D7:C45.1
D8:AOUT+  (via drill 0.6)
  Top 0.406: v30.8,11.75 D8:C43.2 30.16,12.65 D8:U1.4 30.16,15.56 D8:R44.1
  Bottom 0.406: v30.8,11.75 D8:R43.2
D8:AOUT-  (via drill 0.6)
  Top 0.406: D8:R34.1 30.16,18.1 D8:U1.5 30.16,20.64 D8:C33.2 v30.8,21.91
  Bottom 0.406: v30.8,21.91 D8:R33.2
D8:FB+  (via drill 0.6)
  Top 0.406: v21.91,21.91 D8:R32.1 D8:C32.2 D8:R31.2
  Bottom 0.406: D8:R33.1 v21.91,21.91 D8:C32.2
D8:FB-  (via drill 0.6)
  Top 0.406: v21.91,11.75 D8:R42.1 D8:R41.2
  Bottom 0.406: D8:R43.1 v21.91,11.75 D8:C42.2
D8:N$1
  Top 0.406: D8:R34.2 35.24,20.32 D8:C34.2 37.78,20.37 D8:R35.1
D8:N$2  (via drill 0.6)
  Top 0.406: D8:U1.2 27.62,15.56 v26.99,16.19
  Bottom 0.406: v26.99,16.19 25.67,16.51 D8:C7.1
D8:N$3
  Top 0.406: D8:R44.2 35.24,13.34 D8:C44.2 37.78,13.29 D8:R45.1
D8:N$4
  Top 0.406: D8:R42.2 D8:U1.1 26.35,13.02 D8:C43.1
D8:N$5
  Top 0.406: D8:C33.1 26.35,20.64 D8:U1.8 D8:R32.2
D8:N$10
  Top 0.406: D8:R41.1 D8:C41.1
D8:R31
  Top 0.406: D8:C31.1 D8:R31.1
D8:VB+  (via drill 0.6)
  Top 0.406: v19.37,21.91 D8:R36.1
  Bottom 0.406: D8:C35.1 v19.37,21.91 D8:R36.1 D8:R37.2
D8:VB-  (via drill 0.6)
  Top 0.406: D8:R46.2 v19.37,11.75
  Bottom 0.406: D8:R47.1 D8:R46.2 v19.37,11.75 D8:C45.1
GND  (via drill 0.6)
  Top 0.254: U3.15 52.77,110.74 v53.02,110.49 | U3.EXP 50.73,110.24 U3.14 52.77,110.24 v53.02,110.49 | U3.13 52.91,109.74 53.02,109.86 v53.02,110.49 | U3.16 52.91,111.24 53.02,111.12 v53.02,110.49
  Top 0.305: R1.1 39.8,8.58 v39.69,8.46 | C1.2 5.4,110.17 v6.67,110.81
  Top 0.406: D1:U1.6 28.89,111.44 v28.26,110.81 | D1:C34.1 v35.24,110.17 D1:C44.1 | D2:U1.6 28.89,98.11 v28.26,97.47 | D2:C34.1 v35.24,96.84 D2:C44.1 | D3:U1.6 28.89,84.77 v28.26,84.14 | D3:C34.1 v35.24,83.5 D3:C44.1 | D4:U1.6 28.89,71.44 v28.26,70.8 | D4:C34.1 v35.24,70.17 D4:C44.1 | D5:U1.6 28.89,58.1 v28.26,57.47 | D5:C34.1 v35.24,56.83 D5:C44.1 | D6:U1.6 28.89,44.77 v28.26,44.13 | D6:C34.1 v35.24,43.5 D6:C44.1 | D7:U1.6 28.89,31.43 v28.26,30.8 | D7:C34.1 v35.24,30.16 D7:C44.1 | D8:U1.6 28.89,18.1 v28.26,17.46 | D8:C34.1 v35.24,16.83 D8:C44.1 | R7.1 5.67,33.97 v5.67,32.71 | C19.1 20.16,5.94 19.53,6.57 R31.1 | v39.69,8.47 v39.69,8.46 | C5.2 C8.2 v46.04,115.57 | R19.2 57.19,108.31 v57.15,107.63 | C9.2 58.04,114.05 v58.1,113.98 | R15.2 48.67,105.5 v48.58,105.41 | R3.1 11.67,3.73 v11.75,3.81
  Top 0.61: C4.1 v2.21,20.43 | v2.21,20.43 | C20.1 37.17,5.62 T11.TP
  Top 0.813: C19.1 17.03,5.32 X2.2
  Bottom 0.254: v53.02,110.49 53.02,109.86
  Bottom 0.406: v28.26,110.81 26.99,110.81 | v35.24,110.17 35.24,109.54 | v28.26,97.47 26.99,97.47 | v35.24,96.84 35.24,96.2 | v28.26,84.14 26.99,84.14 | v35.24,83.5 35.24,82.87 | v28.26,70.8 26.99,70.8 | v35.24,70.17 35.24,69.53 | v28.26,57.47 26.99,57.47 | v35.24,56.83 35.24,56.2 | v28.26,44.13 26.99,44.13 | v35.24,43.5 35.24,42.86 | v28.26,30.8 26.99,30.8 | v35.24,30.16 35.24,29.53 | v28.26,17.46 26.99,17.46 | v35.24,16.83 35.24,16.19 | v39.69,8.46 39.69,7.83 38.43,6.57 T11.TP | T11.TP | v46.04,115.57 44.45,115.57 | v57.15,107.63 56.83,108.27 56.52,107.95 | v58.1,113.98 59.69,113.98 | v48.58,105.41 50.8,105.41 51.12,105.09 | v11.75,3.81 13.34,3.81 13.97,3.17 | C3.1 17.2,9.59 T9.TP
  Bottom 0.61: v2.21,20.43 1.89,20.43 0.95,21.37
  pour Bottom: 0.95,116.5 10.99,116.5 10.99,2.29 0.95,2.29
  pour Bottom: 11.11,116.5 39.05,116.5 39.05,103.82 11.11,103.82
  pour Bottom: 11.11,103.82 39.05,103.82 39.05,90.49 11.11,90.49
  pour Bottom: 11.11,90.49 39.05,90.49 39.05,77.15 11.11,77.15
  pour Bottom: 11.11,77.15 39.05,77.15 39.05,63.82 11.11,63.82
  pour Bottom: 11.11,63.82 39.05,63.82 39.05,50.48 11.11,50.48
  pour Bottom: 11.11,50.48 39.05,50.48 39.05,37.15 11.11,37.15
  pour Bottom: 11.11,37.15 39.05,37.15 39.05,23.81 11.11,23.81
  pour Bottom: 11.11,23.81 39.05,23.81 39.05,10.48 11.11,10.48
  pour Bottom: 10.4,10.35 26.77,10.35 26.77,2.48 10.4,2.48
  pour Bottom: 35.91,10.48 41.92,10.48 41.92,2.48 35.91,2.48
  pour Bottom: 39.05,98.74 39.05,13.3 63.5,13.3 63.5,98.73
  pour Bottom: 39.05,116.52 63.5,116.52 63.5,98.74 38.42,98.74
HVIN  (via drill 0.6)
  Top 0.254: U3.5 48.26,111.28 v47.62,111.76 U3.4
  Top 0.406: R9.2 42.95,113.9 44.45,112.39 | 44.45,112.39 45.72,112.39 46.04,112.08 47.31,112.08 v47.62,111.76 | R17.1 44.08,112.02 44.45,112.39
  Bottom 0.254: C35.1 v47.62,111.76
  Bottom 0.406: v47.62,111.76 R8.1 HVIN.TP
IN0  (via drill 0.6)
  Top 0.406: D1:C41.2 v13.02,108.9
  Top 0.61: X1.31 3.81,80.01 6.16,80.01 6.16,81.6 6.16,96.46 11.24,101.54 11.24,108.78 11.74,109.24 12.55,109.24 12.56,109.23 v13.02,108.9
  Bottom 0.406: v13.02,108.9 D1:R47.2
IN1  (via drill 0.6)
  Top 0.61: D2:C41.2 v13.02,95.57 12.38,96.71 10.09,96.7 8.7,95.67 8.7,76.64 7.05,75.12 5.4,75.12 X1.27
  Bottom 0.61: v13.02,95.57 13.97,95.57 D2:R47.2
IN2  (via drill 0.6)
  Top 0.406: D3:C41.2 v13.02,82.23
  Top 0.61: X1.23 5.4,70.04 8.32,70.04 10.6,72.33 10.6,81.85 11.62,83.38 12.38,83.38 v13.02,82.23
  Bottom 0.406: v13.02,82.23 D3:R47.2
IN3  (via drill 0.6)
  Top 0.406: D4:C41.2 v13.02,68.9
  Top 0.61: X1.19 5.4,64.96 9.08,64.96 11.62,70.04 12.38,70.04 v13.02,68.9
  Bottom 0.406: v13.02,68.9 D4:R47.2
IN4  (via drill 0.6)
  Top 0.406: D5:C41.2 v13.02,55.56
  Top 0.61: X1.15 9.21,59.37 11.11,56.83 12.38,56.83 v13.02,55.56
  Bottom 0.406: v13.02,55.56 D5:R47.2
IN5  (via drill 0.6)
  Top 0.406: D6:C41.2 v13.02,42.23
  Top 0.61: X1.11 9.21,54.29 11.11,49.85 11.11,44.13 v13.02,42.23
  Bottom 0.406: v13.02,42.23 D6:R47.2
IN6  (via drill 0.6)
  Top 0.61: X1.7 7.94,49.21 9.21,47.94 9.21,33.97 11.75,30.8 12.38,30.16 v13.02,28.89 D7:C41.2
  Bottom 0.61: v13.02,28.89 D7:R47.2
IN7  (via drill 0.6)
  Top 0.406: D8:C41.2 v13.02,15.56
  Top 0.61: X1.3 5.4,44.13 7.05,43.5 7.05,29.78 10.48,26.99 10.48,18.1 v13.02,15.56
  Bottom 0.406: v13.02,15.56 D8:R47.2
IP0  (via drill 0.6)
  Top 0.406: X1.32 1.59,80.33 | D1:C31.2 v13.02,111.44
  Top 0.61: 1.59,80.33 2.22,80.33 2.86,80.96 5.4,80.96 5.4,96.84 10.48,101.92 10.48,109.54 11.43,110.17 12.38,110.17 v13.02,111.44
  Bottom 0.406: v13.02,111.44 D1:R37.1
IP1  (via drill 0.6)
  Top 0.406: D2:C31.2 v13.02,98.11
  Top 0.61: X1.28 2.86,75.88 6.67,75.88 7.94,77.15 7.94,96.2 9.84,97.47 12.38,97.47 v13.02,98.11
  Bottom 0.406: v13.02,98.11 D2:R37.1
IP2  (via drill 0.6)
  Top 0.406: D3:C31.2 v13.02,84.77
  Top 0.61: X1.24 2.86,70.8 7.94,70.8 9.84,72.71 9.84,82.23 11.11,84.14 12.38,84.14 v13.02,84.77
  Bottom 0.406: v13.02,84.77 D3:R37.1
IP3  (via drill 0.6)
  Top 0.406: D4:C31.2 v13.02,71.44
  Top 0.61: X1.20 2.86,65.72 8.57,65.72 11.11,70.8 12.38,70.8 v13.02,71.44
  Bottom 0.406: v13.02,71.44 D4:R37.1
IP4  (via drill 0.6)
  Top 0.406: D5:C31.2 v13.02,58.1
  Top 0.61: X1.16 2.86,60.64 5.4,60.64 6.03,60.13 9.59,60.13 11.49,57.59 12.38,57.59 v13.02,58.1
  Bottom 0.406: v13.02,58.1 D5:R37.1
IP5  (via drill 0.6)
  Top 0.406: D6:C31.2 v13.02,44.77
  Top 0.61: X1.12 2.86,55.56 5.4,55.56 6.03,55.05 9.72,55.05 11.87,50.1 11.87,44.64 12.64,44.26 13.02,44.26 v13.02,44.77
  Bottom 0.406: v13.02,44.77 D6:R37.1
IP6  (via drill 0.6)
  Top 0.61: D7:C31.2 v13.02,31.43 13.02,31.56 12.26,31.56 9.97,34.35 9.97,48.32 8.32,49.97 6.03,49.97 5.4,50.48 2.86,50.48 X1.8
  Bottom 0.61: D7:R37.1 v13.02,31.43
IP7  (via drill 0.6)
  Top 0.406: D8:C31.2 v13.02,18.1
  Top 0.61: X1.4 2.86,45.4 5.4,45.4 7.81,44.13 7.81,30.16 11.24,27.5 11.24,18.48 11.49,18.22 12.38,17.59 v13.02,18.1
  Bottom 0.406: v13.02,18.1 D8:R37.1
LDAC1
  Bottom 0.305: U1.4 4.79,108.75 4.76,110.81 R6.1
  Bottom 0.406: R5.2 6.03,113.03 LDAC1.TP 5.08,111.76 4.76,110.81
LDAC2
  Bottom 0.305: U2.4 4.64,24.96 4.76,25.08 4.76,26.44 4.36,26.44 3.81,26.99 R12.1 5.38,27.61 LDAC2.TP 5.4,29.2 R11.2
N$1  (via drill 0.6)
  Top 0.305: C1.1 5.08,106.05 4.76,105.73 v3.81,105.73 3.81,106.68 4.13,111.44 v2.22,112.71 2.22,114.3 3.17,115.25 R4.1
  Bottom 0.305: U1.1 3.68,106.24 v3.81,105.73
  Bottom 0.406: R6.2 2.84,112.09 v2.22,112.71
N$2
  Top 0.406: R3.2 7.91,6.25 R2.1 6.85,7.62 6.03,7.62 5.08,8.57 3.81,8.57 3.46,8.92 3.46,10.62 IC1.1
N$3
  Top 0.305: LED1.C 41.41,6.67 R1.2
N$4
  Top 0.406: LED2.C 2.1,34.39 R7.2
N$5
  Bottom 0.406: R8.2 46.04,104.46 X3.1
N$7
  Top 0.254: U3.11 50.72,108.35 R15.1 T14.TP
N$9
  Top 0.254: 46.83,110.73 U3.6
  Top 0.305: R17.2 46.83,110.73
N$10
  Bottom 0.305: U4.6 41.62,102.58 42.55,102.23 R13.1
N$11  (via drill 0.6)
  Top 0.61: v3.49,30.8 3.81,30.48 3.81,22.86 v4.13,21.27
  Bottom 0.305: U2.1 4,21.4 v4.13,21.27 | v3.49,30.8 R12.2
  Bottom 0.61: R10.1 v3.49,30.8 | v4.13,21.27 C2.1
N$13
  Top 0.254: U3.1 51.75,112.08 T15.TP
  Bottom 0.254: R16.1 T15.TP
N$20
  Top 0.61: R31.2 23.63,8.46 R30.1 24.89,8.15 25.51,8.78 26.3,8.78 IC2.1
ON0
  Top 0.61: D1:R45.2 40.2,108.58 | 40.2,108.58 | 40.2,108.58 40.2,105.41 43.05,102.55 43.05,96.2 45.91,93.34 45.91,85.38 51.94,79.3 51.94,49.53 53.34,47.94 59.05,47.94 59.69,47.31 59.69,46.99 X5.A12
ON1
  Top 0.61: D2:R45.2 39.05,95.25 40.77,90.49 40.77,85.23 50.29,79.52 50.29,48.28 51.31,46.67 X5.C12
ON2  (via drill 0.6)
  Top 0.61: D3:R45.2 40,81.91 40.01,81.92 46.86,74.93 46.86,42.55 v50.48,39.05
  Route3 0.61: v50.48,39.05 51.75,39.05 53.02,40.32 58.74,40.32 X5.A9
ON3  (via drill 0.6)
  Top 0.61: D4:R45.2 44.13,68.58 44.64,67.94 44.64,41.91 v51.36,35.16
  Route3 0.61: v51.36,35.16 51.36,35.48 X5.C9
ON4  (via drill 0.6)
  Top 0.61: D5:R45.2 40.96,55.24 42.42,53.66 42.42,40.96 51.59,31.75 v53.02,31.75
  Route3 0.61: v53.02,31.75 53.66,32.7 58.74,32.7 X5.A6
ON5  (via drill 0.6)
  Top 0.61: D6:R45.2 39.88,41.91 | 39.88,41.91 | 39.88,41.91 39.88,40.32 v53.02,27.15
  Route3 0.61: v53.02,27.15 53.02,29.53 X5.C6
ON6
  Top 0.61: D7:R45.2 37.78,29.53 39.05,29.53 39.56,28.89 39.56,24.7 40.7,23.81 X5.C3
ON7
  Top 0.61: D8:R45.2 37.78,16.38 58.1,16.38 58.74,17.14 58.74,22.54 X5.A3
OP0  (via drill 0.6)
  Top 0.61: D1:R35.2 37.47,110.49 40.32,110.49 40.96,109.86 40.96,105.73 43.81,102.87 43.81,96.52 46.67,93.66 46.67,85.72 52.7,79.69 52.7,52.07 53.34,51.44 v53.34,50.48
  Route2 0.61: v53.34,50.48 53.02,45.72 53.34,45.4 58.74,45.4 X5.A11
OP1  (via drill 0.6)
  Top 0.61: D2:R35.2 v37.78,96.84 | v37.78,91.12 40.01,88.9 40.01,84.77 49.53,79.06 49.53,47.94 50.8,45.91 53.02,45.91 X5.C11
  Route3 0.61: v37.78,96.84 v37.78,91.12
OP2
  Top 0.61: D3:R35.2 37.78,83.82 39.29,83.82 47.62,75.25 47.62,42.94 50.29,40.32 58.1,40.32 58.74,39.69 58.74,37.78 X5.A8
OP3
  Top 0.61: D4:R35.2 44.13,71.76 45.4,70.48 45.4,42.35 51.22,36.51 X5.C8
OP4
  Top 0.61: D5:R35.2 42.23,58.42 43.18,57.47 43.18,41.27 51.75,32.7 58.1,32.7 58.74,32.07 58.74,29.84 X5.A5
OP5
  Top 0.61: D6:R35.2 40,45.09 40.64,44.45 40.64,40.64 52.39,28.89 X5.C5
OP6
  Top 0.61: D7:R35.2 37.78,30.29 39.43,30.29 40.32,29.34 40.32,25.21 41.08,24.57 53.34,24.57 53.98,25.08 55.88,25.08 56.2,24.77 56.2,22.54 X5.C2
OP7  (via drill 0.6)
  Top 0.61: D8:R35.2 37.78,17.14 55.56,17.14 56.2,17.78 v56.2,20
  Route2 0.61: v56.2,20 58.74,20 X5.A2
PWRGND
  Route2 0.61: X5.A30 X5.B30 X5.C30
  Route3 0.61: X5.B29 X5.B30
  Bottom 0.61: R20.2 52.94,88.19 53.34,88.58 56.2,88.58 X5.B29
SCL  (via drill 0.6)
  Route2 0.305: v1.91,106.68 3.49,107 4.76,107 9.53,106.05 10.48,103.19 37.15,103.19 v37.15,102.23 45.4,102.23 v45.72,101.92 | v2.22,22.22 3.49,23.18 5.4,23.18 6.67,21.91 9.84,21.91 11.11,23.18 37.78,23.18 37.78,22.86 40.32,20.32 41.7,20.32 SCL.TP
  Route3 0.305: v33.66,104.78 33.66,104.46 35.88,102.23 v37.15,102.23 | v45.72,101.92 44.13,100.65 44.13,96.84 44.77,96.2 v44.77,84.77 44.77,80.64 43.44,79.31 SCL.TP
  Bottom 0.305: U1.2 2.2,107.76 1.85,106.98 v1.91,106.68 | U2.2 2.35,23.94 1.59,23.18 1.59,22.54 v2.22,22.22 | U4.5 39.69,101.92 37.47,101.92 v37.15,102.23 | R38.1 34.61,105.73 v33.66,104.78 | U8.2 42.42,85.53 43.18,84.77 43.5,84.77 | 43.5,84.77 v44.77,84.77 | U5.2 43.47,84.75 43.5,84.77
SCLEXT  (via drill 0.6)
  Route2 0.305: X5.C29 50.39,89.85 X4.3 44,89.03 v42.23,88.9
  Bottom 0.305: v42.23,88.9 41.59,88.58 41.2,88.1 U8.3 | R32.1 47.3,90.49 47.31,90.49 47.31,90.17 47.94,89.53 48.75,89.53 X4.3
SDA  (via drill 0.6)
  Route2 0.305: v2.22,110.81 6.67,108.27 10.16,106.68 13.02,103.82 37.15,103.82 v37.47,104.46 38.1,103.5 v45.09,103.5 | v2.22,26.99 2.22,25.08 3.49,23.81 6.03,23.81 7.3,22.54 9.21,22.54 10.48,23.81 39.03,23.81 SDA.TP
  Route3 0.305: v45.09,103.5 42.55,100.97 v42.55,93.66 43.18,93.03 v43.18,81.28 42.55,80.64 42.55,78.42 40.89,76.77 SDA.TP
  Bottom 0.305: U1.3 2.22,108.27 1.96,108.95 v2.22,110.81 | U2.3 2.22,24.45 1.59,25.08 1.59,26.35 v2.22,26.99 | v37.47,104.46 39.05,105.09 R37.1 | U8.7 42.42,93.54 v42.55,93.66 | U5.1 42.84,81.62 v43.18,81.28
  Bottom 0.406: U4.4 37.8,104.13 v37.47,104.46
SDAEXT  (via drill 0.6)
  Route2 0.305: X5.A29 60.01,90.17 59.05,91.12 50.02,91.12 X4.2 43,91.58 v40.64,93.98
  Bottom 0.305: R33.1 50.02,91.12 X4.2 | v40.64,93.98 41.27,93.54 U8.6
V5  (via drill 0.6)
  Top 0.406: D1:U1.3 v28.89,109.54 | D2:U1.3 v28.89,96.2 | D3:U1.3 v28.89,82.87 | D4:U1.3 v28.89,69.53 | D5:U1.3 v28.89,56.2 | D6:U1.3 v28.89,42.86 | D7:U1.3 v28.89,29.53 | D8:U1.3 v28.89,16.19
  Top 0.61: R30.2 IC2.2
  Top 1.016: IC2.2 v29.29,6.26 | v29.29,6.26
  Route3 1.016: v28.89,109.54 28.89,100.01 30.8,97.47 D2:C1.2 v28.89,96.2 28.89,86.68 30.8,84.77 D3:C1.2 v28.89,82.87 28.89,72.71 30.16,72.07 30.23,69.98 v28.89,69.53 28.89,60.01 30.8,58.1 D5:C1.2 v28.89,56.2 28.89,46.67 30.8,44.77 30.8,43.5 v28.89,42.86 28.89,33.97 30.8,32.7 D7:C1.2 v28.89,29.53 28.89,20.64 30.8,18.73 D8:C1.2 v28.89,16.19 28.91,16.18 28.91,9.16 v29.29,8.78
  Bottom 0.406: v28.89,109.54 30.8,110.17 D1:C1.2 D1:C2.2 | v28.89,96.2 30.8,96.84 D2:C1.2 D2:C2.2 | v28.89,82.87 30.8,83.5 D3:C1.2 D3:C2.2 | v28.89,69.53 30.8,70.17 D4:C1.2 D4:C2.2 | v28.89,56.2 30.8,56.83 D5:C1.2 D5:C2.2 | v28.89,42.86 30.8,43.5 D6:C1.2 D6:C2.2 | v28.89,29.53 30.8,30.16 D7:C1.2 D7:C2.2 | v28.89,16.19 30.8,16.83 D8:C1.2 D8:C2.2
  other vias: 32.44,2.79 30.87,3.42 29.29,3.42 31.5,9.09 33.39,8.78 34.02,5.94 29.29,5 29.29,7.52
  pour Bottom (no thermals): 28.35,9.72 28.35,2.48 34.96,2.48 34.96,9.72
  pour Top (no thermals): 28.35,10.04 28.35,2.48 39.37,2.48 39.37,10.04
  pour Route2 (no thermals): 41.91,10.16 41.91,2.48 22.54,2.48 22.54,10.16
V5D  (via drill 0.6)
  Top 0.254: U3.3 50.23,112.64 50.16,112.71 50.16,113.03 C5.1
  Top 0.406: LED2.A 4.2,37.97 3.78,38.39 2.89,38.39 v2.86,38.42 | R2.2 8.57,8.26 8.26,8.57 6.35,8.57 5.36,9.56 5.36,10.41 IC1.2 | v44.13,114.62 45.4,113.67 C8.1 C5.1
  Top 0.61: R4.2 v7.94,115.25 | C4.2 1.58,17.27 0.95,17.91 0.95,37.45 2.21,38.07 2.83,38.39 v2.86,38.42
  Top 1.27: IC1.2 5.67,13.81
  Route2 0.305: v39.37,109.54 v44.13,114.62 | v39.37,98.42 39.37,98.11 40.01,97.47 v45.4,97.47
  Route3 0.305: v42.86,106.05 39.37,103.82 v39.37,98.42 41.27,96.52 41.27,95.25 41.59,94.93 41.59,92.71 41.27,92.39 v41.27,78.74
  Route3 0.406: v7.94,115.25 10.16,116.2 42.55,116.2 v44.13,114.62 | v39.37,109.54 42.23,107.31 v42.86,106.05
  Route3 0.61: v7.94,115.25 8.26,112.71 7.3,103.82 7.3,99.69 2.86,97.47 v2.86,38.42
  Bottom 0.305: v39.37,109.54 39.37,108.27 R37.2 R38.2 | U4.3 38.75,99.05 v39.37,98.42 39.69,98.11 C6.1 | U8.8 44.01,94.81 C18.1 44.13,96.52 45.09,97.47 v45.4,97.47 R14.2 | R13.2 43.18,105.73 v42.86,106.05 | v41.27,78.74 41.35,78.82 U5.8 42.84,77.18 C7.1
  Bottom 0.406: R16.2 45.09,113.67 v44.13,114.62
  Bottom 0.61: R10.2 3.49,37.15 v2.86,38.42
  pour Top (no thermals): 0.95,17.91 8.19,17.91 11.34,14.76 11.34,12.56 0.95,12.56
VBIAS  (via drill 0.6)
  Top 0.254: U3.8 49.08,109.72 v47.94,108.9
  Top 0.406: D1:R36.2 v13.02,114.62 | v13.02,101.28 D2:R36.2 | D3:R36.2 v13.02,87.95 | D8:R36.2 v13.02,21.27 | v13.02,34.61 D7:R36.2 | v13.02,47.94 D6:R36.2 | v13.02,61.28 D5:R36.2 | v13.02,74.61 D4:R36.2 | R9.1 40.02,112 VB.TP
  Route3 0.406: v13.02,114.62 14.29,114.62 | 14.29,114.62 D2:R36.2 | D2:R36.2 v13.02,101.28 | v13.02,87.95 D3:R36.2 | D3:R36.2 14.92,87.95 14.92,100.97 D2:R36.2 | v13.02,21.27 14.92,21.27 14.92,34.29 D7:R36.2 | D7:R36.2 v13.02,34.61 | D7:R36.2 D6:R36.2 | D6:R36.2 v13.02,47.94 | D6:R36.2 D5:R36.2 | D5:R36.2 v13.02,61.28 | D5:R36.2 D4:R36.2 | D4:R36.2 v13.02,74.61 | D4:R36.2 D3:R36.2 | 14.29,114.62 16.51,114.62 17.14,114.3 29.84,114.3 31.75,112.39 39.62,112.39 VB.TP 42.47,109.54 44.77,109.54 45.4,108.9 v47.94,108.9
VEXT  (via drill 0.6)
  Route2 0.61: v51.75,97.47 X5.C32
  Route3 0.61: X5.C32 X5.B32 X5.A32 | X4.1 49.66,94.11 51.75,96.2 v51.75,97.47
  Bottom 0.305: X4.1 51.3,94.11 R33.2
  Bottom 0.406: R32.2 47.3,92.39 47.62,92.71 48.17,92.71 X4.1
  Bottom 0.61: v51.75,97.47 R14.1
VEXT2
  Route2 0.61: X5.C31 X5.B31 X5.A31
VIN+
  Top 0.813: 26.3,3.9 IC2.3
  Top 1.016: 14.18,3.11 19.85,3.11
  Top 1.27: IC1.3 7.98,10.69 | 7.98,10.69 T4.TP 14.17,5.01 X2.1 14.17,4.39 14.18,3.11 | 7.98,10.69 | 19.85,3.11 C19.2 22.99,3.1 23.62,3.9 26.3,3.9
  Bottom 0.406: C3.2 11.17,9.59 T4.TP
VTR1  (via drill 0.6)
  Top 0.305: v12.8,105.74 D1:R48.1
  Route2 0.305: v9.43,111.13 11.18,108.89 10.79,108.65 10.79,108.59 v12.8,105.74
  Bottom 0.305: U1.6 7.49,109.89 v9.43,111.13
VTR2  (via drill 0.6)
  Top 0.305: v12.38,92.39 D2:R48.1
  Route3 0.305: v9.21,109.54 10.79,109.22 10.86,107.07 10.86,94.39 v12.38,92.39
  Bottom 0.305: U1.7 8.76,108.78 v9.21,109.54
VTR3  (via drill 0.6)
  Top 0.305: v13.02,79.06 D3:R48.1
  Route3 0.305: v9.53,107.95 9.53,107.3 9.53,98.1 8.26,96.52 8.26,80.01 9.84,79.06 v13.02,79.06
  Bottom 0.305: U1.8 8.57,108.27 v9.53,107.95
VTR4  (via drill 0.6)
  Top 0.305: v13.02,65.72 D4:R48.1
  Route2 0.305: v6.99,66.99 11.75,66.99 v13.02,65.72
  Route3 0.305: v8.57,105.09 8.57,99.38 6.67,96.2 5.72,95.57 5.4,68.58 v6.99,66.99
  Bottom 0.305: U1.9 6.16,107.76 6.03,107.63 6.03,105.09 v8.57,105.09
VTR5  (via drill 0.6)
  Top 0.305: v13.02,52.39 D5:R48.1
  Route3 0.305: v7.3,26.99 7.3,30.16 9.59,31.75 9.59,51.18 10.79,52.39 v13.02,52.39
  Bottom 0.305: U2.6 v7.3,26.99
VTR6  (via drill 0.6)
  Top 0.305: v13.02,39.05 D6:R48.1
  Route3 0.305: v8.57,26.35 8.57,28.26 11.1,29.52 11.1,33.33 11.11,34.61 11.11,39.05 v13.02,39.05
  Bottom 0.305: U2.7 8.45,24.96 8.57,25.08 v8.57,26.35
VTR7  (via drill 0.6)
  Top 0.305: v13.02,25.72 D7:R48.1
  Route2 0.305: v9.21,24.45 11.75,24.45 v13.02,25.72
  Bottom 0.305: U2.8 v9.21,24.45
VTR8  (via drill 0.6)
  Top 0.305: v11.75,12.38 D8:R48.1
  Route3 0.305: v9.5,20.32 9.81,17.78 9.81,16.92 11.66,15.07 v11.75,12.38
  Bottom 0.305: U2.9 6.16,23.94 6.03,23.81 6.03,22.59 6.93,22 v9.5,20.32

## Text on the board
Top: comp
Route2: route1
Route3: route3
Bottom: bottom
tNames: SERIALNR: | Universiteit Antwerpen | SOLID Amplifier V2.0.1 / 20150921 / W.Beaumont
bNames: SOLID Amplifier V2.0.1 / 20150921 / W.Beaumont / Universiteit Antwerpen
